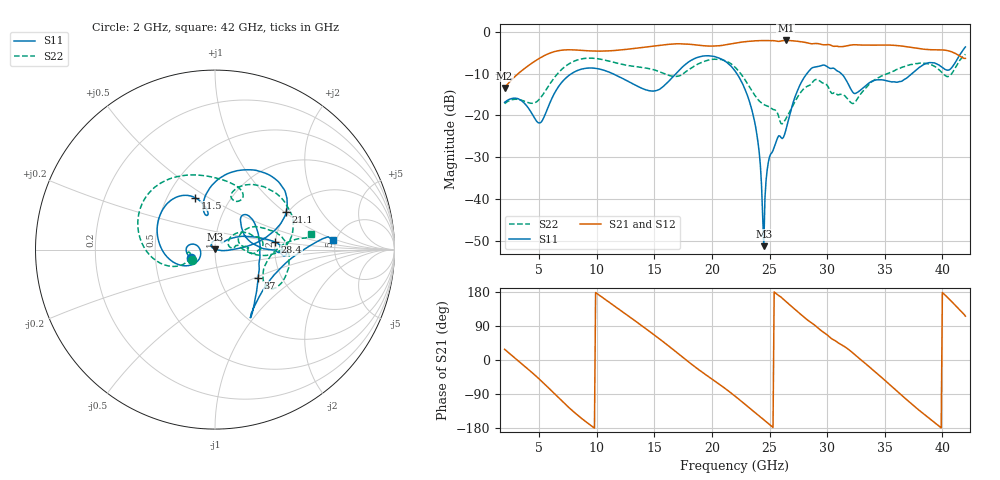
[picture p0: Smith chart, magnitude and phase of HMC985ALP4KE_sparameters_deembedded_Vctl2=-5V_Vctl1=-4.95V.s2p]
!s2p File: Measurements: S11, S21, S12, S22
# GHz S dB R 50.0
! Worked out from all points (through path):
!   401 points, 2 GHz to 42 GHz, reference 50 ohm
!   highest |S21| = -2.06 dB at 26.4 GHz (marker M1); lowest = -13.4 dB at 2 GHz (marker M2)
!   lowest |S11| = -51.3 dB at 24.5 GHz (marker M3), VSWR 1.01, Z = 49.9 + j0.246 ohm
!   |S11| at or under -10 dB: start of sweep to 7.81 GHz; 22.16 GHz to 28.24 GHz (6.081 GHz wide, 24.1 % of centre); 31.23 GHz to 37.36 GHz (6.138 GHz wide, 17.9 % of centre)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
!   |S22| runs from -22.0 to -5.4 dB; largest |S21 - S12| = 0.0011
!   S11 on the Smith chart (normalised r, x): 2 GHz: 0.76, -0.07; 11.5 GHz: 0.68, +0.44; 21.1 GHz: 1.96, +1.03; 28.4 GHz: 1.99, +0.19; 37 GHz: 1.52, -0.52; 42 GHz: 4.70, +0.86
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2  -16.88 -161.7  -13.43 28.3  -13.43 28.3  -17.19 -155.5
5  -21.82 -172.3  -6.37 -50.1  -6.37 -50.1  -16.18 -159.6
6.3  -14.84 -150.2  -4.76 -88.3  -4.76 -88.3  -11.03 -161.4
8.7  -8.91 150.4  -4.44 -154.5  -4.44 -154.5  -6.46 151.4
11.5  -10.16 111.2  -4.47 143.2  -4.48 143.3  -7.31 105.2
13.6  -13.11 101.2  -3.86 97.3  -3.86 97.3  -8.40 75.8
15.4  -13.82 105.8  -3.26 56.6  -3.26 56.7  -9.49 62.2
17.9  -7.34 80.4  -2.95 -3.3  -2.95 -3.3  -9.21 72.2
21.1  -6.96 27.8  -3.15 -74.1  -3.15 -74.1  -6.86 16.3
22  -9.34 17.2  -2.71 -95.3  -2.72 -95.3  -8.45 0.8
23.6  -20.19 0.1  -2.18 -135.0  -2.18 -134.9  -14.70 -4.3
24.5  -51.30 115.0  -2.08 -157.6  -2.08 -157.6  -17.39 8.0
25  -29.89 133.4  -2.11 -170.3  -2.11 -170.3  -17.97 10.8
26.4  -23.64 41.8  -2.06 155.0  -2.06 155.0  -20.88 33.2
28.4  -9.45 7.3  -2.72 103.1  -2.72 103.1  -12.87 18.8
28.7  -8.62 2.3  -2.86 96.8  -2.86 96.9  -12.19 16.8
30.7  -8.96 -2.7  -3.45 50.9  -3.45 51.0  -14.59 2.7
32.5  -14.69 31.5  -3.10 11.4  -3.10 11.4  -16.54 27.5
35.4  -11.83 19.5  -3.17 -64.2  -3.17 -64.1  -9.83 19.6
37  -10.85 -33.1  -3.59 -107.3  -3.60 -107.2  -8.03 5.4
39.8  -8.12 -57.2  -4.31 -176.6  -4.31 -176.6  -9.29 -35.3
42  -3.62 4.5  -6.34 115.7  -6.35 115.8  -5.37 9.0
